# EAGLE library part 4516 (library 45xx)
Binary up down COUNTER
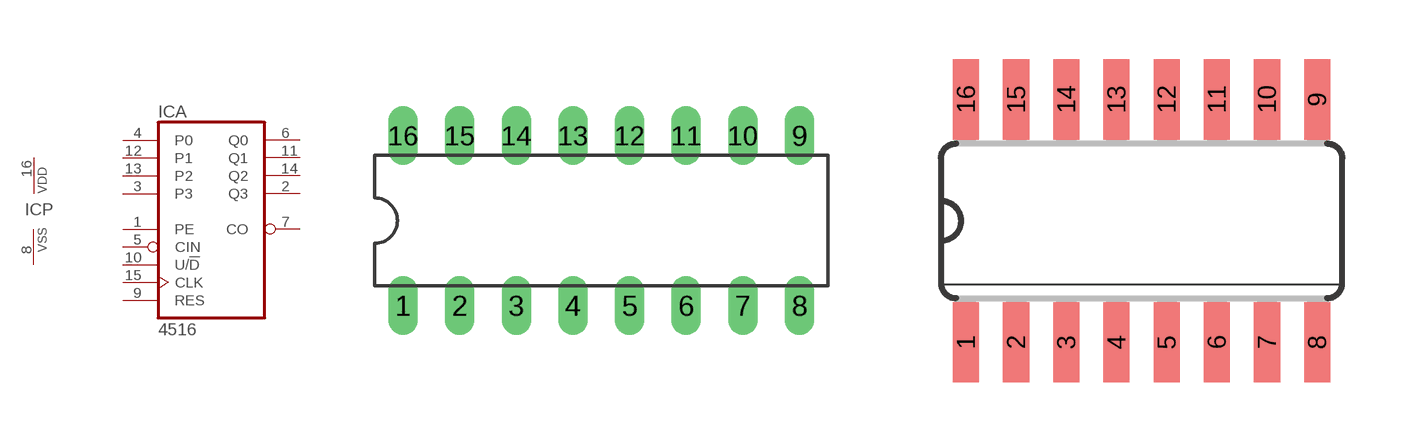
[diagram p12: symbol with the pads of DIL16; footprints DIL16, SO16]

Designator prefix IC; gates A=4516 P=PWRN

## 4516N  [DIL16]
1  A:PE  in
2  A:Q3  out
3  A:P3  in
4  A:P0  in
5  A:CIN  in
6  A:Q0  out
7  A:CO  out
8  P:VSS  pwr
9  A:RES  in
10  A:U/!D  in
11  A:Q1  out
12  A:P1  in
13  A:P2  in
14  A:Q2  out
15  A:CLK  in
16  P:VDD  pwr

## 4516D  [SO16]
Pads as for DIL16

## Footprint DIL16 (pad centres in mm)
Dual In Line Package
drill 0.813 long: 1 -8.89,-3.81; 2 -6.35,-3.81; 3 -3.81,-3.81; 4 -1.27,-3.81; 5 1.27,-3.81; 6 3.81,-3.81; 7 6.35,-3.81; 8 8.89,-3.81; 9 8.89,3.81; 10 6.35,3.81; 11 3.81,3.81; 12 1.27,3.81; 13 -1.27,3.81; 14 -3.81,3.81; 15 -6.35,3.81; 16 -8.89,3.81

## Footprint SO16 (pad centres in mm)
Small Outline package 150 mil
smd 0.66 x 2.032: 1 -4.445,-3.073; 2 -3.175,-3.073; 3 -1.905,-3.073; 4 -0.635,-3.073; 5 0.635,-3.073; 6 1.905,-3.073; 7 3.175,-3.073; 8 4.445,-3.073; 9 4.445,3.073; 10 3.175,3.073; 11 1.905,3.073; 12 0.635,3.073; 13 -0.635,3.073; 14 -1.905,3.073; 15 -3.175,3.073; 16 -4.445,3.073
